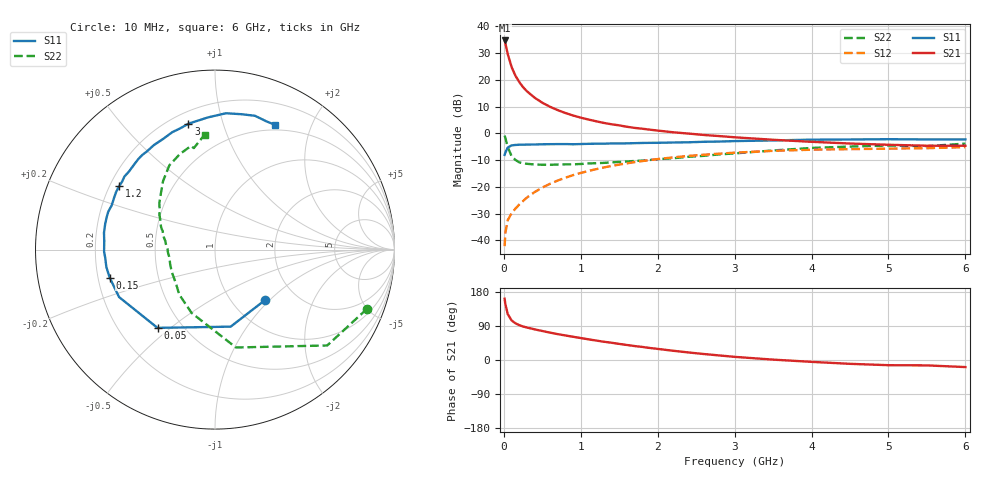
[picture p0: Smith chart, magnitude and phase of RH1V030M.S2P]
! SIEMENS Small Signal Semiconductors
! BFR106
! Si NPN RF Bipolar Junction Transistor in SOT23
! VCE = 1 V  IC = 30 mA
! Common Emitter S-Parameters:  August  1996
# GHz  S  MA  R  50
!  f  S11  S21  S12  S22
! GHz  MAG  ANG  MAG  ANG  MAG  ANG  MAG  ANG
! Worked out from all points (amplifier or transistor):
!   36 points, 10 MHz to 6 GHz, reference 50 ohm
!   highest |S21| = 34.7 dB at 10 MHz (marker M1)
!   |S21| within 3 dB of that: start of sweep to 34.63 MHz
!   unconditionally stable (mu >= 1): 265.7 MHz to 3.848 GHz; 4.046 GHz to end of sweep
!   at 250 MHz: K = 0.99, MSG = 21.3 dB, |S12| = -25.3 dB
!   at 1.4 GHz: K = 1.08, MAG = 6.1 dB, |S12| = -12.2 dB
!   at 6 GHz: K = 1.02, MAG = -0.6 dB, |S12| = -5.2 dB
!   S11 on the Smith chart (normalised r, x): 10 MHz: 1.42, -0.94; 50 MHz: 0.37, -0.45; 150 MHz: 0.25, -0.12; 1.2 GHz: 0.24, +0.29; 3 GHz: 0.27, +0.78; 6 GHz: 0.44, +1.50
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0.01  0.3963 -44.9  54.45 161.7  0.0078 76.5  0.909 -21.3
0.02  0.438 -78.5  48.05 147.3  0.0139 66.6  0.8224 -40.5
0.05  0.5411 -126.3  30.59 121.4  0.0238 51.7  0.5578 -77.9
0.1  0.5964 -153.7  17.5 104.6  0.032 51.5  0.3762 -110.3
0.15  0.6072 -165.1  11.98 96.9  0.0392 54.7  0.3199 -128.5
0.2  0.6131 -170.9  9.132 92.1  0.0467 58.5  0.2875 -139.3
0.25  0.6132 -175.6  7.304 88.4  0.0545 60.8  0.2748 -148.3
0.3  0.618 -178.9  6.123 85.7  0.0632 63.1  0.2699 -153.7
0.4  0.6191 175.5  4.642 80.9  0.08 65.0  0.2624 -162.2
0.5  0.6257 171.3  3.736 76.5  0.097 65.7  0.2589 -167.9
0.6  0.6283 166.8  3.14 72.3  0.1141 65.5  0.2585 -171.5
0.7  0.63 163.4  2.72 68.2  0.1312 64.9  0.2617 -174.9
0.9  0.6261 156.7  2.157 61.3  0.1658 62.6  0.2641 178.8
1.1  0.6376 149.9  1.813 54.6  0.1985 60.0  0.2736 174.8
1.2  0.6404 146.5  1.682 51.3  0.2143 58.3  0.2773 172.3
1.7  0.6563 132.4  1.266 36.8  0.2895 50.1  0.3049 162.1
2.2  0.6748 120.2  1.049 24.4  0.3557 41.3  0.3425 152.3
3  0.7169 101.9  0.845 8.3  0.4355 27.7  0.4221 136.3
3.5  0.7374 93.1  0.759 1.0  0.4713 20.0  0.4789 127.2
4.5  0.7685 79.0  0.646 -10.1  0.5072 6.1  0.567 110.2
5.5  0.7699 68.1  0.587 -14.2  0.5287 -2.1  0.5777 101.8
6  0.7713 64.2  0.586 -18.7  0.5518 -8.7  0.6435 95.1
